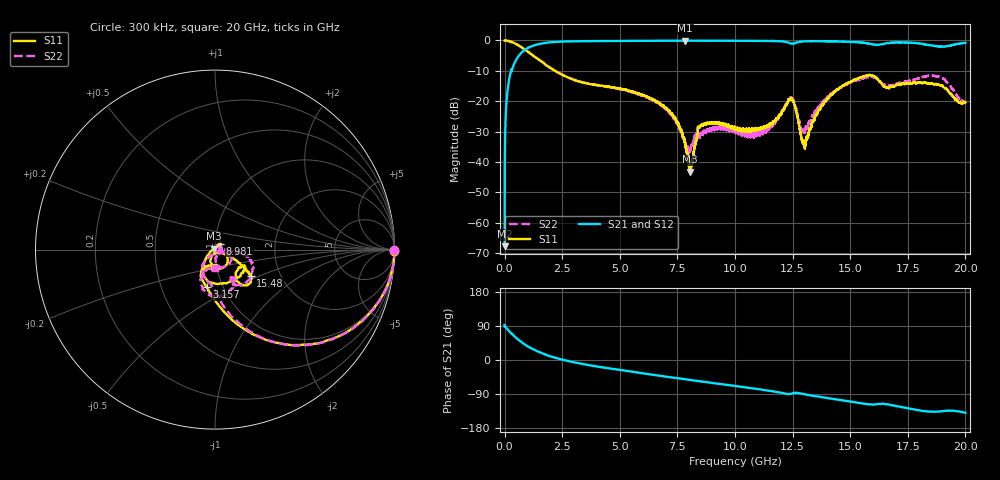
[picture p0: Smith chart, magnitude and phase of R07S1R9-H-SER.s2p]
!{R07S1R9}
!Johanson Technology Inc.
!www.johansontechnology.com
!Test Board Conditions:
!Substrate Type  RO4350B
!Substrate Thickness  10 mil
!Substrate Dk  3.66
!TL Type: GCPW
!TL Trace Width  21 mil
!TL Gap  20 mil
!Electrode orientation  Horizontal
!DUT TOPOLOGY	SERIES
!Mounting Pad LxW  16x21 mil
! Created Sat Feb  6 11:25:40 2021
# hz S ma R 50
! 2 Port Network Data from SP1.SP block
! freq  magS11  angS11  magS21  angS21  magS12  angS12  magS22  angS22
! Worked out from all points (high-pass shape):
!   20001 points, 300 kHz to 20 GHz, reference 50 ohm
!   highest |S21| = -0.06 dB at 7.836 GHz (marker M1); lowest = -67.7 dB at 300 kHz (marker M2)
!   |S21| within 3 dB of the highest: 884.3 MHz to end of sweep
!   lowest |S11| = -43.1 dB at 8.051 GHz (marker M3), VSWR 1.01, Z = 49.5 + j0.45 ohm
!   |S11| at or under -10 dB: 2.192 GHz to end of sweep
!   |S22| runs from -36.9 to 0.0 dB; largest |S21 - S12| = 0.011
!   S11 on the Smith chart (normalised r, x): 300 kHz: open; 3.157 GHz: 0.84, -0.37; 8.981 GHz: 1.06, +0.07; 15.48 GHz: 1.42, -0.44; 20 GHz: 0.97, -0.19
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300000  0.998 -0.3  0.0004128 92.2  0.0004317 89.0  0.9975 -0.2
1.013e8  0.9914 -7.4  0.1203 82.8  0.1203 82.8  0.9909 -7.4
1.323e8  0.9871 -9.7  0.1564 80.5  0.1563 80.6  0.9867 -9.8
4.803e8  0.883 -29.8  0.4629 59.8  0.4629 59.6  0.8835 -30.0
1.5333e9  0.4678 -70.2  0.878 20.3  0.8793 20.2  0.4724 -68.5
3.1573e9  0.2148 -102.4  0.973 -7.7  0.9727 -7.8  0.2181 -91.8
3.3343e9  0.2064 -104.9  0.9742 -9.9  0.9739 -9.9  0.2087 -93.6
6.6673e9  0.09537 -129.4  0.9881 -40.9  0.9886 -41.0  0.09236 -130.7
7.8363e9  0.01981 -163.9  0.9929 -50.8  0.9905 -50.9  0.02188 -96.2
8.0513e9  0.006966 139.2  0.99 -52.6  0.9913 -52.6  0.01553 -49.2
8.4813e9  0.03831 50.1  0.9899 -56.2  0.9889 -56.2  0.02734 14.2
8.9813e9  0.04398 50.2  0.9869 -60.2  0.9891 -60.2  0.03397 1.9
1.00003e10  0.03635 26.2  0.9871 -68.5  0.9883 -68.5  0.03093 1.3
1.12703e10  0.03803 -20.1  0.9846 -79.3  0.9852 -79.3  0.03303 18.8
1.24123e10  0.1099 -65.6  0.8898 -89.6  0.8898 -89.6  0.1165 -46.9
1.29733e10  0.02057 -74.5  0.968 -90.1  0.967 -90.0  0.03231 -46.2
1.33343e10  0.04204 -24.2  0.9736 -93.8  0.974 -94.0  0.05443 -16.1
1.42033e10  0.1279 -27.5  0.9663 -101.7  0.9641 -102.0  0.1324 -8.2
1.54773e10  0.2477 -36.5  0.9236 -114.0  0.9209 -114.1  0.2366 -25.0
1.66673e10  0.1649 -37.5  0.9015 -117.2  0.9055 -117.6  0.1794 -58.2
1.87853e10  0.1891 -90.0  0.803 -136.1  0.8 -136.2  0.2553 -95.1
2e10  0.09667 -93.3  0.9161 -139.2  0.912 -139.1  0.1016 -87.7
